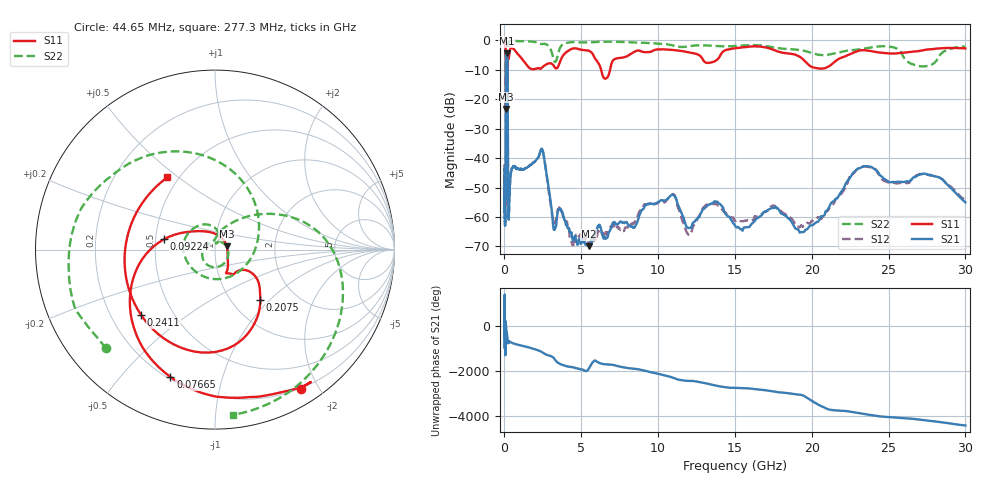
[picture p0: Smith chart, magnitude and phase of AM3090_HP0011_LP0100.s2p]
! Date/Time: Thu, Feb 28, 2019 1:56 PM
! Network Analyzer: Agilent Technologies E8364B Rev: A.07.50.67
! Sweep from 0.010 to 30.000 GHz, 1601 Points, Sweep Type: LOG
! Power Supply: 5.023 V, 0.002 A
# Hz S DB R 50
!freq MagS11 AngS11 MagS21 AngS21 MagS12 AngS12 MagS22 AngS22
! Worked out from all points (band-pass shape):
!   1601 points, 10 MHz to 30 GHz, reference 50 ohm
!   highest |S21| = -4.48 dB at 145.4 MHz (marker M1); lowest = -69.9 dB at 5.473 GHz (marker M2)
!   |S21| within 3 dB of the highest: 101.9 MHz to 196.6 MHz (94.66 MHz wide, 63.4 % of centre)
!   lowest |S11| = -23.4 dB at 100.4 MHz (marker M3), VSWR 1.15, Z = 56.9 + j2.09 ohm
!   |S11| at or under -10 dB: 91.76 MHz to 199.8 MHz (108.1 MHz wide, 74.1 % of centre); 6.288 GHz to 6.877 GHz (588.6 MHz wide, 8.94 % of centre)
!   |S22| runs from -29.3 to -0.1 dB; largest |S21 - S12| = 0.014
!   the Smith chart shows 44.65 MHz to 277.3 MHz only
!   S11 on the Smith chart (normalised r, x): 44.65 MHz: 0.19, -1.77; 76.65 MHz: 0.21, -0.69; 92.24 MHz: 0.55, +0.07; 207.5 MHz: 1.35, -0.88; 241.1 MHz: 0.33, -0.34; 277.3 MHz: 0.44, +0.46
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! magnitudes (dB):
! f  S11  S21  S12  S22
! 10 MHz  -0.2  -43.5  -42.8  -0.5
! 38.04 MHz  -0.5  -61.0  -62.9  -1.3
! 44.65 MHz  -0.8  -58.0  -57.0  -1.7
! 76.65 MHz  -2.5  -46.8  -47.0  -4.7
! 92.24 MHz  -10.7  -15.4  -15.4  -15.6
! 100.4 MHz  -23.4  -8.0  -8.0  -15.1
! 144.7 MHz  -15.8  -4.5  -4.4  -23.1
! 145.4 MHz  -15.7  -4.5  -4.4  -22.8
! 185.8 MHz  -14.0  -5.9  -5.9  -26.8
! 207.5 MHz  -8.5  -11.5  -11.5  -12.9
! 241.1 MHz  -5.2  -54.0  -55.6  -1.6
! 277.3 MHz  -6.3  -60.6  -57.3  -0.7
! 550.5 MHz  -2.9  -43.0  -42.8  -0.2
! 2.084 GHz  -9.7  -40.6  -40.5  -0.8
! 2.507 GHz  -9.1  -37.9  -37.8  -1.3
! 3.236 GHz  -9.0  -63.9  -61.6  -7.2
! 5.473 GHz  -3.6  -69.9  -69.1  -0.8
! 7.926 GHz  -5.6  -61.6  -63.6  -0.7
! 10.76 GHz  -3.3  -53.1  -53.1  -1.6
! 19.61 GHz  -7.5  -64.2  -62.2  -3.8
! 23.48 GHz  -3.5  -42.8  -42.9  -2.9
! 30 GHz  -2.8  -55.0  -54.4  -2.2
